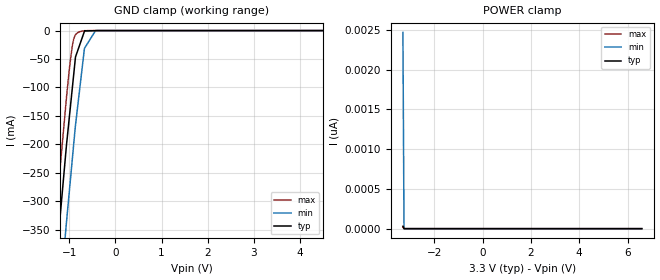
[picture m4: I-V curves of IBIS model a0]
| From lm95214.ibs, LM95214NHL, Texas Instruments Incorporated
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[Model]   a0
Model_type   Input
Vinl = 0.33
Vinh = 2.97
|   typ   min   max
|   (nom PVT)   (fast PVT)   (slow PVT)
C_comp   0.380p   0.356p   0.409p
[Model spec]
|subparameter
Vinl   0.33   0.3   0.36
Vinh   2.97   2.70   3.24
[Voltage Range]   3.3   3   3.6
[Temperature Range]   27   125   -40
[Power Clamp Reference]   3.3   3   3.6
[GND Clamp Reference]   0   0   0
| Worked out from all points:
|   GND clamp passes 1 mA (typ) near -0.67 V on its own axis
[GND Clamp]
|   Voltage   I(typ)   I(min)   I(max)
-3.3V     -2.347A    -2.466A    -2.274A
-1.457V   -567.9mA   -705.1mA   -481.5mA
-1.267V   -388.2mA   -525.4mA   -301.6mA
-1.259V   -380.6mA   -517.9mA   -293.9mA
-1.069V   -207mA     -342.4mA   -123.4mA
-986.8mV  -141.2mA   -270.3mA   -57.96mA
-912.6mV  -82.4mA    -205.3mA   -17.2mA
-867.1mV  -46.34mA   -166.2mA   -7.369mA
-770.3mV  -23.82mA   -98.83mA   -1.77mA
-673.2mV  -1.235mA   -31.33mA   -232.4uA
-431.7mV  -135.5uA   0A         -14.27uA
6.59V     0A         0A         0A
[POWER Clamp]
|   Voltage   I(typ)   I(min)   I(max)
-3.3V     30.41pA    2.468nA    20.74pA
-3.254V   267.9fA    0A         356.8fA
-3.253V   0A         0A         0A
6.59V     0A         0A         0A
